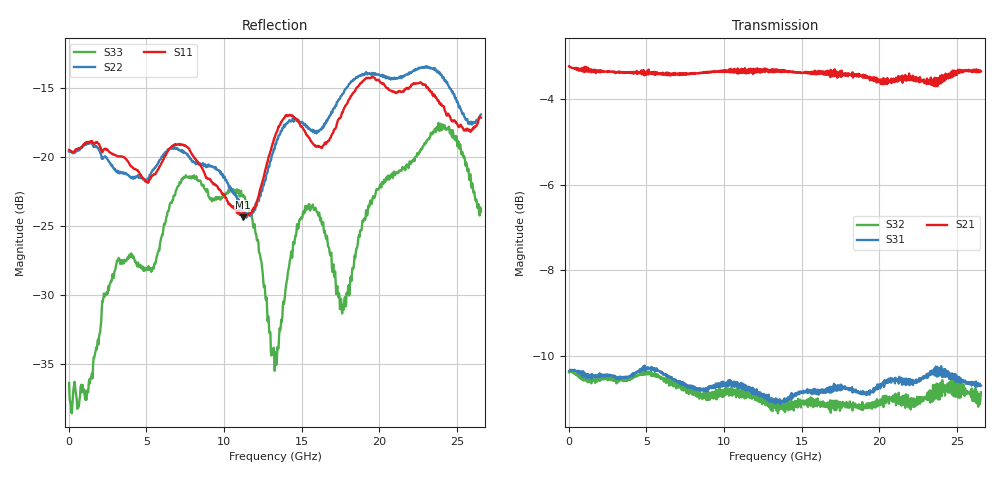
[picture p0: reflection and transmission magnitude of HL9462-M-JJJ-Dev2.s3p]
! 4/7/2020 11:11:52 AM
! H:\PRODUCTION_DATA\TEMP_S3P.S3P
! CHANNEL.1
! TR.MEASUREMENT
! CORRECTED.DATA
# GHZ S RI R 50.0
! FREQ.GHZ  S11RE  S11IM  S12RE  S12IM  S13RE  S13IM
!  S21RE  S21IM  S22RE  S22IM  S23RE  S23IM
!  S31RE  S31IM  S32RE  S32IM  S33RE  S33IM
!; PortSelection: Port_123
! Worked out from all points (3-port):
!   758 points, 35 MHz to 26.53 GHz, reference 50 ohm
!   strongest paths, dB at 35 MHz, 6.65 GHz, 13.3 GHz, 19.91 GHz, 26.53 GHz:
!     S21: -3.2, -3.4, -3.3, -3.5, -3.4
!     S31: -10.4, -10.5, -11.1, -10.8, -10.7
!     S32: -10.4, -10.6, -11.0, -11.1, -10.8
!   lowest |S11| = -24.4 dB at 11.2 GHz (marker M1), VSWR 1.13, Z = 51.7 - j5.93 ohm
!   |S11| at or under -10 dB: start of sweep to end of sweep
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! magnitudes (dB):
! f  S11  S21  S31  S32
! 35 MHz  -19.5  -3.2  -10.4  -10.4
! 3.15 GHz  -19.9  -3.4  -10.5  -10.5
! 7.35 GHz  -19.1  -3.4  -10.6  -10.7
! 11.2 GHz  -24.4  -3.4  -10.6  -10.9
! 13.3 GHz  -18.4  -3.3  -11.1  -11.0
! 15.33 GHz  -18.4  -3.4  -10.8  -11.0
! 17.64 GHz  -16.8  -3.4  -10.7  -11.1
! 19.84 GHz  -14.4  -3.6  -10.8  -11.0
! 23.73 GHz  -15.9  -3.7  -10.3  -10.8
! 26.53 GHz  -17.1  -3.4  -10.7  -10.8
